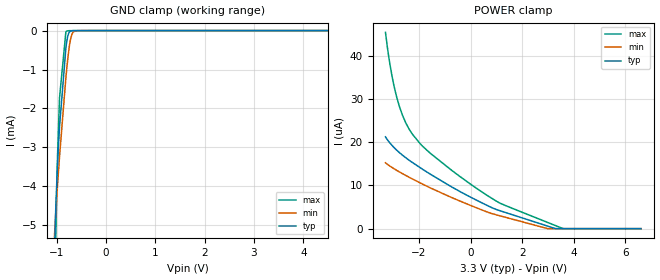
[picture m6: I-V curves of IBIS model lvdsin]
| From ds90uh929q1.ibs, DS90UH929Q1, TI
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|   Model
[Model]   lvdsin
Model_type   Input
Vinl = 2.8
Vinh = 2.9
|   typ   min   max
C_comp   0.121pF   0.088pF   0.152pF
[Voltage Range]   3.3   3   3.6
[Temperature Range]   27   105   -40
[Power Clamp Reference]   3.3   3   3.6
[GND Clamp Reference]   0   0   0
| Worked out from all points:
|   GND clamp passes 1 mA (typ) near -0.85 V on its own axis
[GND Clamp]
|   Voltage   I(typ)   I(min)   I(max)
-3.3V     -329.2mA   -303.5mA   -349.4mA
-1.043V   -5.545mA   -5.193mA   -7.219mA
-1.023V   -4.681mA   -4.746mA   -5.607mA
-1.013V   -4.311mA   -4.537mA   -4.899mA
-983.4mV  -3.391mA   -3.95mA    -3.183mA
-943.8mV  -2.465mA   -3.232mA   -1.724mA
-815.1mV  -450.4uA   -1.211mA   -32.27uA
-795.3mV  -267.7uA   -950.7uA   -12.43uA
-745.8mV  -42.64uA   -413uA     -2.894uA
-706.2mV  -8.071uA   -151uA     -2.06uA
-597.3mV  -1.299uA   -3.963uA   -1.557uA
6.6V      0A         0A         0A
[POWER Clamp]
|   Voltage   I(typ)   I(min)   I(max)
-3.3V     21.27uA    15.27uA    45.46uA
-3.142V   19.95uA    14.55uA    38.58uA
-2.963V   18.75uA    13.86uA    32.9uA
-2.765V   17.64uA    13.16uA    28.4uA
-2.528V   16.49uA    12.37uA    24.69uA
-2.27V    15.38uA    11.55uA    21.98uA
-1.954V   14.11uA    10.59uA    19.66uA
-815.1mV  9.947uA    7.415uA    13.89uA
1.125V    4.177uA    2.988uA    5.947uA
2.977V    601.7nA    15.86nA    1.454uA
3.58V     0A         0A         5.547nA
6.6V      0A         0A         0A
